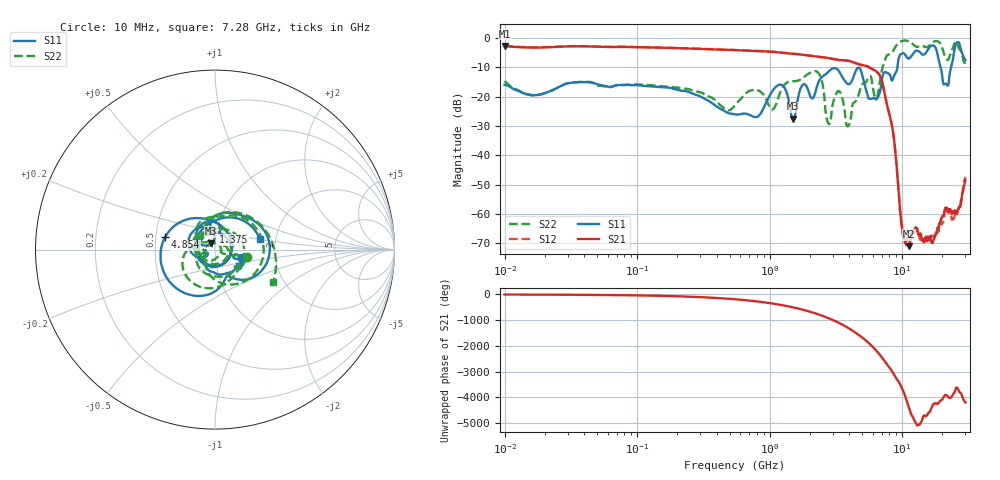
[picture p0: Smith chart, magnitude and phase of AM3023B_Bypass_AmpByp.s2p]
# Hz S DB R 50.0
!freq dBS11 angS11 dBS21 angS21 dBS12 angS12 dBS22 angS22
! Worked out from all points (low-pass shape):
!   1601 points, 10 MHz to 30 GHz, reference 50 ohm
!   highest |S21| = -2.80 dB at 10 MHz (marker M1); lowest = -70.9 dB at 11.19 GHz (marker M2)
!   |S21| within 3 dB of the highest: start of sweep to 1.811 GHz
!   lowest |S11| = -27.6 dB at 1.505 GHz (marker M3), VSWR 1.09, Z = 47.5 + j3.26 ohm
!   |S11| at or under -10 dB: start of sweep to 9.206 GHz; 19.48 GHz to 23.4 GHz (3.915 GHz wide, 18.3 % of centre)
!   |S22| runs from -30.1 to -0.9 dB; largest |S21 - S12| = 0.019
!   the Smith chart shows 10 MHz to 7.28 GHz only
!   S11 on the Smith chart (normalised r, x): 10 MHz: 1.35, -0.12; 1.375 GHz: 0.96, +0.19; 4.854 GHz: 0.56, +0.09; 7.28 GHz: 1.65, +0.21
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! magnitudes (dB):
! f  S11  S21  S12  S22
! 10 MHz  -16.0  -2.8  -2.7  -14.7
! 38.04 MHz  -15.1  -2.9  -2.8  -15.0
! 144.7 MHz  -16.7  -3.3  -3.3  -16.4
! 547.7 MHz  -26.0  -4.2  -4.1  -23.0
! 1.375 GHz  -20.1  -5.3  -5.3  -15.0
! 1.505 GHz  -27.6  -5.4  -5.4  -14.8
! 1.775 GHz  -16.0  -5.7  -5.7  -13.7
! 2.084 GHz  -20.6  -6.2  -6.2  -11.6
! 2.785 GHz  -11.5  -6.9  -6.9  -29.3
! 3.318 GHz  -11.2  -7.5  -7.5  -18.1
! 3.934 GHz  -15.8  -7.8  -7.8  -29.9
! 4.854 GHz  -10.9  -9.2  -9.1  -16.9
! 5.783 GHz  -20.8  -10.4  -10.3  -13.1
! 6.391 GHz  -20.9  -11.4  -11.4  -20.5
! 7.28 GHz  -11.8  -17.7  -17.7  -8.6
! 7.926 GHz  -12.2  -25.2  -25.1  -5.7
! 10.08 GHz  -5.3  -66.1  -66.6  -1.0
! 11.19 GHz  -7.1  -70.9  -69.5  -1.2
! 17.3 GHz  -2.7  -68.8  -67.8  -1.3
! 21.45 GHz  -15.6  -57.9  -58.3  -6.9
! 25.82 GHz  -1.7  -59.1  -58.9  -1.5
! 30 GHz  -7.6  -48.5  -47.3  -9.1
